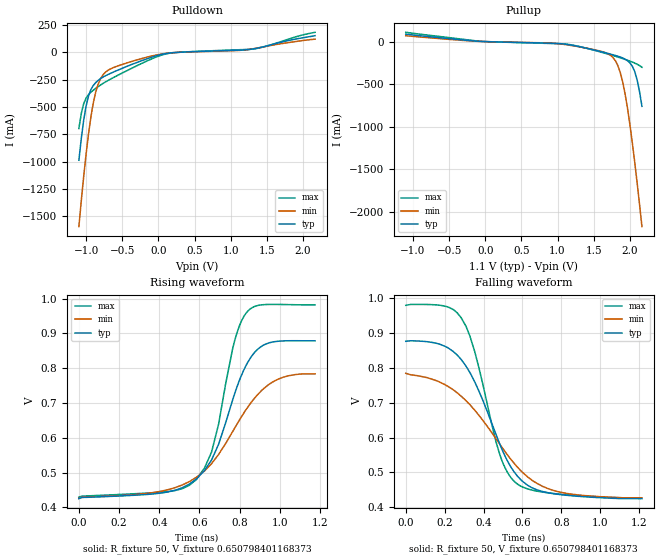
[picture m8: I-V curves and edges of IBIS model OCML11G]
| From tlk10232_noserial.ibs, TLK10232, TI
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[Model]   OCML11G
Model_type   Output
Polarity   Non-Inverting
Cref =  15.0000pF
Rref =  100.0000M
Vref =  0V
Vmeas =  0.66
C_comp   0   0   0
[Temperature Range]   25   125   -40
[Voltage Range]   1.1   0.99   1.21
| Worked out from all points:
|   slope of the pulldown table from 0 to 0.165 V, typ, clamps not added: 7.98 ohm
|   slope of the pullup table from 0 to 0.165 V, typ, clamps not added: 42 ohm
|   rising waveform, R_fixture 50, V_fixture 0.650798401168373: 20-80 % time 179ps typ, 262ps min, 126ps max; typ from 0.425 V to 0.879 V
|   falling waveform, R_fixture 50, V_fixture 0.650798401168373: 20-80 % time 211ps typ, 307ps min, 150ps max; typ from 0.877 V to 0.424 V
[Pulldown]
-1.1V     -987.4mA   -1.594A    -696.9mA
-1.067V   -788.3mA   -1.357A    -559.3mA
-1.033V   -620.6mA   -1.134A    -469.9mA
-1V       -490.4mA   -929.4mA   -418.1mA
-933.3mV  -340.2mA   -589mA     -364.7mA
-900mV    -302.6mA   -460.8mA   -346.2mA
-833.3mV  -256.6mA   -290.7mA   -313.8mA
-733.3mV  -214.8mA   -182.7mA   -271.5mA
-433.3mV  -128.1mA   -96.7mA    -166.9mA
100mV     -11.76mA   -9.882mA   -15.5mA
1.333V    33.71mA    35.05mA    32.39mA
2.167V    152mA      120.4mA    183.1mA
[Pullup]
-1.1V     88.16mA    69.53mA    109.8mA
-66.67mV  3.14mA     2.495mA    4.434mA
1V        -21.58mA   -23.55mA   -24.03mA
1.533V    -103.5mA   -99.97mA   -107.5mA
1.733V    -146.8mA   -161.2mA   -155.5mA
1.833V    -171.3mA   -281.6mA   -181.3mA
1.9V      -191.6mA   -472.4mA   -199.4mA
1.933V    -205.6mA   -612.4mA   -208.8mA
2V        -249.2mA   -973.1mA   -228.9mA
2.067V    -351.2mA   -1.415A    -251.8mA
2.1V      -448.8mA   -1.657A    -265.2mA
2.167V    -760.1mA   -2.172A    -300.9mA
[Ramp]
dV/dt_f   0.49482/0.2273981n  0.4225252/0.3244918n  0.5591725/0.1632801n
dV/dt_r  0.4945406/0.2251578n  0.4223491/0.3083486n  0.5589015/0.1630925n
R_load = 53
[Rising Waveform]
R_fixture = 50
V_fixture = 0.650798401168373
V_fixture_min = 0.605273215856304
V_fixture_max = 0.704507758555187
0s        424.9mV    425.8mV    429mV
375ps     438.8mV    442.8mV    442.3mV
550ps     467mV      474.2mV    463.4mV
625ps     505.7mV    504.5mV    513.1mV
660ps     536.1mV    525.4mV    558.7mV
695ps     581.2mV    552mV      638.8mV
765ps     708.8mV    617.7mV    856.1mV
825ps     799.9mV    675mV      952.7mV
940ps     871.5mV    750.9mV    983mV
1.175ns   878.7mV    783.6mV    981.8mV
[Falling Waveform]
R_fixture = 50
V_fixture = 0.650798401168373
V_fixture_min = 0.605273215856304
V_fixture_max = 0.704507758555187
0s        876.7mV    784.7mV    980mV
175ps     868.3mV    759.4mV    980.2mV
285ps     824.6mV    719mV      944.4mV
355ps     759.8mV    678.5mV    846.6mV
485ps     579.5mV    580mV      549.1mV
525ps     531mV      548.9mV    498.4mV
570ps     492.4mV    517.9mV    468.4mV
650ps     455.6mV    477.1mV    448.9mV
780ps     437.1mV    444.9mV    438mV
1.215ns   424.4mV    426.9mV    427mV
